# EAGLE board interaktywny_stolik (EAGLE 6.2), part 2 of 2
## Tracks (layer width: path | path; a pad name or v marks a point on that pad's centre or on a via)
0V
  Bottom 0.406: IC1.10 18.34,221.93 18.34,220.46 | 18.34,220.46 20.85,220.46 20.85,220.48 | 20.85,220.48 IC1.12 | IC1.5 18.34,216.1 18.34,220.46 | IC1.1 IC1.2 | IC1.2 22.07,216.1 22.07,220.48 20.85,220.48 | R6.2 20.96,211.69 20.96,214.41 22.12,214.41 IC1.2
0V1
  Bottom 0.406: IC2.10 98.34,221.93 98.34,220.46 | 98.34,220.46 100.85,220.46 100.85,220.48 | 100.85,220.48 IC2.12 | IC2.5 98.34,216.1 98.34,220.46 | IC2.1 IC2.2 | IC2.2 102.07,216.1 102.07,220.48 100.85,220.48 | R18.2 100.96,211.69 100.96,214.41 102.12,214.41 IC2.2
0V2
  Bottom 0.406: IC3.10 178.34,221.93 178.34,220.46 | 178.34,220.46 180.85,220.46 180.85,220.48 | 180.85,220.48 IC3.12 | IC3.5 178.34,216.1 178.34,220.46 | IC3.1 IC3.2 | IC3.2 182.07,216.1 182.07,220.48 180.85,220.48 | R30.2 180.96,211.69 180.96,214.41 182.12,214.41 IC3.2
0V3
  Bottom 0.406: IC4.10 18.34,141.93 18.34,140.46 | 18.34,140.46 20.85,140.46 20.85,140.48 | 20.85,140.48 IC4.12 | IC4.5 18.34,136.1 18.34,140.46 | IC4.1 IC4.2 | IC4.2 22.07,136.1 22.07,140.48 20.85,140.48 | R42.2 20.96,131.69 20.96,134.41 22.12,134.41 IC4.2
0V4
  Bottom 0.406: IC5.10 98.34,141.93 98.34,140.46 | 98.34,140.46 100.85,140.46 100.85,140.48 | 100.85,140.48 IC5.12 | IC5.5 98.34,136.1 98.34,140.46 | IC5.1 IC5.2 | IC5.2 102.07,136.1 102.07,140.48 100.85,140.48 | R54.2 100.96,131.69 100.96,134.41 102.12,134.41 IC5.2
0V5
  Bottom 0.406: IC6.10 178.34,141.93 178.34,140.46 | 178.34,140.46 180.85,140.46 180.85,140.48 | 180.85,140.48 IC6.12 | IC6.5 178.34,136.1 178.34,140.46 | IC6.1 IC6.2 | IC6.2 182.07,136.1 182.07,140.48 180.85,140.48 | R66.2 180.96,131.69 180.96,134.41 182.12,134.41 IC6.2
0V6
  Bottom 0.406: IC7.10 18.34,61.93 18.34,60.46 | 18.34,60.46 20.85,60.46 20.85,60.48 | 20.85,60.48 IC7.12 | IC7.5 18.34,56.1 18.34,60.46 | IC7.1 IC7.2 | IC7.2 22.07,56.1 22.07,60.48 20.85,60.48 | R78.2 20.96,51.69 20.96,54.41 22.12,54.41 IC7.2
0V7
  Bottom 0.406: IC8.10 98.34,61.93 98.34,60.46 | 98.34,60.46 100.85,60.46 100.85,60.48 | 100.85,60.48 IC8.12 | IC8.5 98.34,56.1 98.34,60.46 | IC8.1 IC8.2 | IC8.2 102.07,56.1 102.07,60.48 100.85,60.48 | R90.2 100.96,51.69 100.96,54.41 102.12,54.41 IC8.2
0V8
  Bottom 0.406: IC9.10 178.34,61.93 178.34,60.46 | 178.34,60.46 180.85,60.46 180.85,60.48 | 180.85,60.48 IC9.12 | IC9.5 178.34,56.1 178.34,60.46 | IC9.1 IC9.2 | IC9.2 182.07,56.1 182.07,60.48 180.85,60.48 | R102.2 180.96,51.69 180.96,54.41 182.12,54.41 IC9.2
GND  (via drill 0.6 pad 0.81)
  Top 0.406: v19.63,223.99 9.5,223.99 v9.47,223.96
  Top 0.813: v35.2,223.91 19.76,223.91 v19.63,223.96
  Bottom 0.406: IC1.11 19.63,221.93 19.63,222.06 | 19.61,224.01 v19.63,223.99
  Bottom 0.813: 40.95,203.39 41.02,203.39 41.02,220.58 35.2,220.58 v35.2,223.91 | v19.63,223.96 19.61,224.01 IC1.11
  Bottom 1.016: R2.1 9.47,223.83 v9.47,223.96 9.47,229.07 11.43,229.07 LED6.K | LED21.K 41,203.41 | 40.97,203.41 40.97,203.57 41,203.57 41,203.41 | 41,203.41 40.97,203.41 | 40.97,203.41 40.97,203.24 40.95,203.24 40.95,203.39
GND1  (via drill 0.6 pad 0.81)
  Top 0.406: v99.63,223.99 89.5,223.99 v89.47,223.96
  Top 0.813: v115.2,223.91 99.76,223.91 v99.63,223.96
  Bottom 0.406: IC2.11 99.63,221.93 99.63,222.06 | 99.61,224.01 v99.63,223.99
  Bottom 0.813: 120.95,203.39 121.02,203.39 121.02,220.58 115.2,220.58 v115.2,223.91 | v99.63,223.96 99.61,224.01 IC2.11
  Bottom 1.016: R14.1 89.47,223.83 v89.47,223.96 89.47,229.07 91.43,229.07 LED34.K | LED28.K 121,203.41 | 120.97,203.41 120.97,203.57 121,203.57 121,203.41 | 121,203.41 120.97,203.41 | 120.97,203.41 120.97,203.24 120.95,203.24 120.95,203.39
GND2  (via drill 0.6 pad 0.81)
  Top 0.406: v179.63,223.99 169.5,223.99 v169.47,223.96
  Top 0.813: v195.2,223.91 179.76,223.91 v179.63,223.96
  Bottom 0.406: IC3.11 179.63,221.93 179.63,222.06 | 179.61,224.01 v179.63,223.99
  Bottom 0.813: 200.95,203.39 201.02,203.39 201.02,220.58 195.2,220.58 v195.2,223.91 | v179.63,223.96 179.61,224.01 IC3.11
  Bottom 1.016: R26.1 169.47,223.83 v169.47,223.96 169.47,229.07 171.43,229.07 LED51.K | LED45.K 201,203.41 | 200.97,203.41 200.97,203.57 201,203.57 201,203.41 | 201,203.41 200.97,203.41 | 200.97,203.41 200.97,203.24 200.95,203.24 200.95,203.39
GND3  (via drill 0.6 pad 0.81)
  Top 0.406: v19.63,143.99 9.5,143.99 v9.47,143.96
  Top 0.813: v35.2,143.91 19.76,143.91 v19.63,143.96
  Bottom 0.406: IC4.11 19.63,141.93 19.63,142.06 | 19.61,144.01 v19.63,143.99
  Bottom 0.813: 40.95,123.39 41.02,123.39 41.02,140.58 35.2,140.58 v35.2,143.91 | v19.63,143.96 19.61,144.01 IC4.11
  Bottom 1.016: R38.1 9.47,143.83 v9.47,143.96 9.47,149.07 11.43,149.07 LED68.K | LED62.K 41,123.41 | 40.97,123.41 40.97,123.57 41,123.57 41,123.41 | 41,123.41 40.97,123.41 | 40.97,123.41 40.97,123.24 40.95,123.24 40.95,123.39
GND4  (via drill 0.6 pad 0.81)
  Top 0.406: v99.63,143.99 89.5,143.99 v89.47,143.96
  Top 0.813: v115.2,143.91 99.76,143.91 v99.63,143.96
  Bottom 0.406: IC5.11 99.63,141.93 99.63,142.06 | 99.61,144.01 v99.63,143.99
  Bottom 0.813: 120.95,123.39 121.02,123.39 121.02,140.58 115.2,140.58 v115.2,143.91 | v99.63,143.96 99.61,144.01 IC5.11
  Bottom 1.016: R50.1 89.47,143.83 v89.47,143.96 89.47,149.07 91.43,149.07 LED85.K | LED79.K 121,123.41 | 120.97,123.41 120.97,123.57 121,123.57 121,123.41 | 121,123.41 120.97,123.41 | 120.97,123.41 120.97,123.24 120.95,123.24 120.95,123.39
GND5  (via drill 0.6 pad 0.81)
  Top 0.406: v179.63,143.99 169.5,143.99 v169.47,143.96
  Top 0.813: v195.2,143.91 179.76,143.91 v179.63,143.96
  Bottom 0.406: IC6.11 179.63,141.93 179.63,142.06 | 179.61,144.01 v179.63,143.99
  Bottom 0.813: 200.95,123.39 201.02,123.39 201.02,140.58 195.2,140.58 v195.2,143.91 | v179.63,143.96 179.61,144.01 IC6.11
  Bottom 1.016: R62.1 169.47,143.83 v169.47,143.96 169.47,149.07 171.43,149.07 LED102.K | LED96.K 201,123.41 | 200.97,123.41 200.97,123.57 201,123.57 201,123.41 | 201,123.41 200.97,123.41 | 200.97,123.41 200.97,123.24 200.95,123.24 200.95,123.39
GND6  (via drill 0.6 pad 0.81)
  Top 0.406: v19.63,63.99 9.5,63.99 v9.47,63.96
  Top 0.813: v35.2,63.91 19.76,63.91 v19.63,63.96
  Bottom 0.406: IC7.11 19.63,61.93 19.63,62.06 | 19.61,64.01 v19.63,63.99
  Bottom 0.813: 40.95,43.39 41.02,43.39 41.02,60.58 35.2,60.58 v35.2,63.91 | v19.63,63.96 19.61,64.01 IC7.11
  Bottom 1.016: R74.1 9.47,63.83 v9.47,63.96 9.47,69.07 11.43,69.07 LED119.K | LED113.K 41,43.41 | 40.97,43.41 40.97,43.57 41,43.57 41,43.41 | 41,43.41 40.97,43.41 | 40.97,43.41 40.97,43.24 40.95,43.24 40.95,43.39
GND7  (via drill 0.6 pad 0.81)
  Top 0.406: v99.63,63.99 89.5,63.99 v89.47,63.96
  Top 0.813: v115.2,63.91 99.76,63.91 v99.63,63.96
  Bottom 0.406: IC8.11 99.63,61.93 99.63,62.06 | 99.61,64.01 v99.63,63.99
  Bottom 0.813: 120.95,43.39 121.02,43.39 121.02,60.58 115.2,60.58 v115.2,63.91 | v99.63,63.96 99.61,64.01 IC8.11
  Bottom 1.016: R86.1 89.47,63.83 v89.47,63.96 89.47,69.07 91.43,69.07 LED136.K | LED130.K 121,43.41 | 120.97,43.41 120.97,43.57 121,43.57 121,43.41 | 121,43.41 120.97,43.41 | 120.97,43.41 120.97,43.24 120.95,43.24 120.95,43.39
GND8  (via drill 0.6 pad 0.81)
  Top 0.406: v179.63,63.99 169.5,63.99 v169.47,63.96
  Top 0.813: v195.2,63.91 179.76,63.91 v179.63,63.96
  Bottom 0.406: IC9.11 179.63,61.93 179.63,62.06 | 179.61,64.01 v179.63,63.99
  Bottom 0.813: 200.95,43.39 201.02,43.39 201.02,60.58 195.2,60.58 v195.2,63.91 | v179.63,63.96 179.61,64.01 IC9.11
  Bottom 1.016: R98.1 169.47,63.83 v169.47,63.96 169.47,69.07 171.43,69.07 LED153.K | LED147.K 201,43.41 | 200.97,43.41 200.97,43.57 201,43.57 201,43.41 | 201,43.41 200.97,43.41 | 200.97,43.41 200.97,43.24 200.95,43.24 200.95,43.39
N$1  (via drill 0.6 pad 0.81)
  Top 0.406: v19.66,213.95 v13.31,213.95
  Bottom 0.406: 9.73,217.1 9.73,217.26 R1.1 12.73,213.95 v13.31,213.95 | IC1.3 20.83,216.1 20.83,216.16 20.85,216.16 20.85,215.15 20.63,215.15 19.71,214.23 19.71,214.01 v19.66,213.95
  Bottom 1.016: R2.2 R1.1
N$2
  Bottom 0.406: IC1.6 17.04,213.9 18.09,213.9 18.09,211.47 R3.2 17.42,211.47 17.4,205.57 25.35,205.6 25.37,211.47 23.67,211.44 R4.1
N$3
  Bottom 0.406: R3.1 14.53,213.14 15.8,213.14 15.8,216.1 IC1.7 15.77,216.11 11.48,216.11 11.48,224.06 R7.2
N$4  (via drill 0.6 pad 0.81)
  Top 0.813: v24.97,198.82 36.32,198.82 v36.32,198.84
  Bottom 0.406: R6.1 20.88,208.62 R4.2 23.47,208.62 23.47,208.37 | 22.45,208.82 22.35,208.82 22.35,213.62 26.11,213.62 26.11,204 24.92,204 24.92,198.79
  Bottom 0.813: 24.92,198.79 24.97,198.79 v24.97,198.82 | v36.32,198.84 38.46,198.84 T1.E
  Bottom 1.016: T1.E 38.56,198.82 38.56,198.66 | R4.2 20.9,208.75 20.9,208.82 22.45,208.82
N$5
  Bottom 1.016: R5.2 41,194.93 T1.C
N$6
  Bottom 0.406: R8.1 17.04,217.84 IC1.9 17.04,223.96 18.24,223.96 18.24,225.66 C2.2
N$7
  Bottom 0.406: R8.2 13.39,220.69 13.39,220 15.85,220 15.85,221.93 IC1.8 15.75,221.93 C1.2 15.72,225.66 15.72,227.16 20.14,227.16 20.14,230.52 24.64,230.52 R10.2
N$8
  Bottom 0.406: R10.1 21.74,229.02 R11.2 22.12,225.69 IC1.13
N$9
  Bottom 1.016: R7.1 13.21,226.91 13.21,228.66 C1.1 C2.1
N$10
  Bottom 0.406: IC1.14 23.42,221.93 23.42,225.69 R11.1
  Bottom 0.61: 55.22,235.57 30.15,235.57 30.15,228.64 27.23,228.64 27.23,225.56 24.59,225.56 R11.1
  Bottom 0.813: R12.2 55.22,195.51 55.22,235.57
N$11
  Bottom 0.61: 30.4,194.42 30.18,194.42 30.18,187.21
  Bottom 1.016: 31.42,210.7 LED1.A 31.6,210.7 31.6,204.35 30.4,204.35 30.4,194.42 | 30.18,187.21 31.42,187.21 LED20.K
N$12
  Bottom 0.61: 31.32,215.02 30.15,215.02 30.15,208.04
  Bottom 1.016: LED2.K 31.32,230.74 31.32,215.02 | 30.15,208.04 28.9,208.04 LED11.A
N$13
  Bottom 1.016: LED3.A 27.31,190.69 27.31,210.35 28.91,210.35 LED1.K
N$14
  Bottom 1.016: LED4.K 4.9,170.7 4.9,232.9 28.92,232.9 LED2.A
N$15
  Bottom 0.61: 11.38,193.91 10.19,193.91 10.19,186.12
  Bottom 1.016: LED5.K 11.38,210.72 11.38,193.91 | 10.19,186.12 11.47,186.12 LED4.A
N$16
  Bottom 1.016: LED3.K 7.01,190.59 7.01,230.72 LED6.A
N$17
  Bottom 1.016: R13.2 38.48,206.87 LED21.A
N$18  (via drill 0.6 pad 0.81)
  Top 0.406: v99.66,213.95 v93.31,213.95
  Bottom 0.406: 89.73,217.1 89.73,217.26 R9.1 92.73,213.95 v93.31,213.95 | IC2.3 100.83,216.1 100.83,216.16 100.85,216.16 100.85,215.15 100.63,215.15 99.71,214.23 99.71,214.01 v99.66,213.95
  Bottom 1.016: R14.2 R9.1
N$19
  Bottom 0.406: IC2.6 97.04,213.9 98.09,213.9 98.09,211.47 R15.2 97.42,211.47 97.4,205.57 105.35,205.6 105.37,211.47 103.67,211.44 R16.1
N$20
  Bottom 0.406: R15.1 94.53,213.14 95.8,213.14 95.8,216.1 IC2.7 95.77,216.11 91.48,216.11 91.48,224.06 R19.2
N$21  (via drill 0.6 pad 0.81)
  Top 0.813: v104.97,198.82 116.32,198.82 v116.32,198.84
  Bottom 0.406: R18.1 100.88,208.62 R16.2 103.47,208.62 103.47,208.37 | 102.45,208.82 102.35,208.82 102.35,213.62 106.11,213.62 106.11,204 104.92,204 104.92,198.79
  Bottom 0.813: 104.92,198.79 104.97,198.79 v104.97,198.82 | v116.32,198.84 118.46,198.84 T2.E
  Bottom 1.016: T2.E 118.56,198.82 118.56,198.66 | R16.2 100.9,208.75 100.9,208.82 102.45,208.82
N$22
  Bottom 0.61: 50.44,229.04 50.27,229.04 50.27,232.67
  Bottom 1.016: LED12.A 48.69,210.75 48.69,213.17 50.44,213.17 50.44,229.04 | 50.27,232.67 50.47,232.67 50.47,233.51 33.25,233.51 33.25,214.77 33.35,214.77 33.35,203.13 32.61,203.13 32.61,202.65 32.06,202.65 32.06,190.56 31.44,190.56 LED11.K
N$23
  Bottom 0.61: 51.16,193.43 50.19,193.43 50.19,187.74
  Bottom 1.016: LED12.K 51.16,210.75 51.16,193.43 | 50.19,187.74 51.47,187.74 LED13.A
N$24
  Bottom 1.016: LED13.K 48.9,170.68 48.9,166.51 74.96,166.51 74.96,232.5 68.93,232.5 LED14.A
N$25
  Bottom 1.016: LED14.K 73.46,230.74 73.46,190.66 71.46,190.66 LED15.A
N$26
  Bottom 1.016: LED16.A 68.94,190.72 LED15.K 68.92,195.51 R12.1
N$27
  Bottom 0.61: 71.5,186.67 70.23,186.67 70.23,193.2
  Bottom 1.016: 71.48,210.7 LED17.A 71.45,193.2 70.23,193.2 | LED16.K 71.5,170.75 71.5,186.67
N$28
  Bottom 0.61: 49.96,173.72 50.22,173.72 50.22,167.68 67.44,167.68 67.49,203.26
  Bottom 1.016: LED18.A 48.77,190.69 48.77,185.35 49.96,185.35 49.96,173.72 | 67.49,203.26 68.91,203.34 LED17.K
N$29
  Bottom 1.016: 51.44,230.69 LED19.A 53.14,230.69 53.14,190.84 51.44,190.84 LED18.K
N$30
  Bottom 1.016: LED20.A 28.75,170.75 28.75,168.46 46.69,168.46 46.69,215.61 48.92,215.61 LED19.K
N$31
  Bottom 1.016: R17.2 121,194.93 T2.C
N$32
  Bottom 0.406: R20.1 97.04,217.84 IC2.9 97.04,223.96 98.24,223.96 98.24,225.66 C4.2
N$33
  Bottom 0.406: R20.2 93.39,220.69 93.39,220 95.85,220 95.85,221.93 IC2.8 95.75,221.93 C3.2 95.72,225.66 95.72,227.16 100.14,227.16 100.14,230.52 104.64,230.52 R21.2
N$34
  Bottom 1.016: R19.1 93.21,226.91 93.21,228.66 C3.1 C4.1
N$35
  Bottom 0.406: R21.1 101.74,229.02 R22.2 102.12,225.69 IC2.13
N$36
  Bottom 0.406: IC2.14 103.42,221.93 103.42,225.69 R22.1
  Bottom 0.61: 135.22,235.57 110.15,235.57 110.15,228.64 107.23,228.64 107.23,225.56 104.59,225.56 R22.1
  Bottom 0.813: R23.2 135.22,195.51 135.22,235.57
N$37
  Bottom 0.61: 130.44,229.04 130.27,229.04 130.27,232.67
  Bottom 1.016: LED8.A 128.69,210.75 128.69,213.17 130.44,213.17 130.44,229.04 | 130.27,232.67 130.47,232.67 130.47,233.51 113.25,233.51 113.25,214.77 113.35,214.77 113.35,203.13 112.61,203.13 112.61,202.65 112.06,202.65 112.06,190.56 111.44,190.56 LED7.K
N$38
  Bottom 0.61: 131.16,193.43 130.19,193.43 130.19,187.74
  Bottom 1.016: LED8.K 131.16,210.75 131.16,193.43 | 130.19,187.74 131.47,187.74 LED9.A
N$39
  Bottom 1.016: LED9.K 128.9,170.68 128.9,166.51 154.96,166.51 154.96,232.5 148.93,232.5 LED10.A
N$40
  Bottom 1.016: LED10.K 153.46,230.74 153.46,190.66 151.46,190.66 LED22.A
N$41
  Bottom 1.016: LED23.A 148.94,190.72 LED22.K R23.1
N$42
  Bottom 0.61: 151.5,186.67 150.23,186.67 150.23,193.2
  Bottom 1.016: 151.48,210.7 LED24.A 151.45,193.2 150.23,193.2 | LED23.K 151.5,170.75 151.5,186.67
N$43
  Bottom 0.61: 129.96,173.72 130.22,173.72 130.22,167.68 147.44,167.68 147.49,203.26
  Bottom 1.016: LED25.A 128.77,190.69 128.77,185.35 129.96,185.35 129.96,173.72 | 147.49,203.26 148.91,203.34 LED24.K
N$44
  Bottom 1.016: 131.44,230.69 LED26.A 133.14,230.69 133.14,190.84 131.44,190.84 LED25.K
N$45
  Bottom 1.016: LED27.A 108.75,170.75 108.75,168.46 126.69,168.46 126.69,215.61 128.92,215.61 LED26.K
N$46
  Bottom 0.61: 110.4,194.42 110.18,194.42 110.18,187.21
  Bottom 1.016: 111.42,210.7 LED29.A 111.6,210.7 111.6,204.35 110.4,204.35 110.4,194.42 | 110.18,187.21 111.42,187.21 LED27.K
N$47
  Bottom 0.61: 111.32,215.02 110.15,215.02 110.15,208.04
  Bottom 1.016: LED30.K 111.32,230.74 111.32,215.02 | 110.15,208.04 108.9,208.04 LED7.A
N$48
  Bottom 1.016: LED31.A 107.31,190.69 107.31,210.35 108.91,210.35 LED29.K
N$49
  Bottom 1.016: LED32.K 84.9,170.7 84.9,232.9 108.92,232.9 LED30.A
N$50
  Bottom 0.61: 91.38,193.91 90.19,193.91 90.19,186.12
  Bottom 1.016: LED33.K 91.38,210.72 91.38,193.91 | 90.19,186.12 91.47,186.12 LED32.A
N$51
  Bottom 1.016: LED31.K 87.01,190.59 87.01,230.72 LED34.A
N$52
  Bottom 1.016: R24.2 118.48,206.87 LED28.A
N$53  (via drill 0.6 pad 0.81)
  Top 0.406: v179.66,213.95 v173.31,213.95
  Bottom 0.406: 169.73,217.1 169.73,217.26 R25.1 172.73,213.95 v173.31,213.95 | IC3.3 180.83,216.1 180.83,216.16 180.85,216.16 180.85,215.15 180.63,215.15 179.71,214.23 179.71,214.01 v179.66,213.95
  Bottom 1.016: R26.2 R25.1
N$54
  Bottom 0.406: IC3.6 177.04,213.9 178.09,213.9 178.09,211.47 R27.2 177.42,211.47 177.4,205.57 185.35,205.6 185.37,211.47 183.67,211.44 R28.1
N$55
  Bottom 0.406: R27.1 174.53,213.14 175.8,213.14 175.8,216.1 IC3.7 175.77,216.11 171.48,216.11 171.48,224.06 R31.2
N$56  (via drill 0.6 pad 0.81)
  Top 0.813: v184.97,198.82 196.32,198.82 v196.32,198.84
  Bottom 0.406: R30.1 180.88,208.62 R28.2 183.47,208.62 183.47,208.37 | 182.45,208.82 182.35,208.82 182.35,213.62 186.11,213.62 186.11,204 184.92,204 184.92,198.79
  Bottom 0.813: 184.92,198.79 184.97,198.79 v184.97,198.82 | v196.32,198.84 198.46,198.84 T3.E
  Bottom 1.016: T3.E 198.56,198.82 198.56,198.66 | R28.2 180.9,208.75 180.9,208.82 182.45,208.82
N$57
  Bottom 1.016: R29.2 201,194.93 T3.C
N$58
  Bottom 0.406: R32.1 177.04,217.84 IC3.9 177.04,223.96 178.24,223.96 178.24,225.66 C6.2
N$59
  Bottom 0.406: R32.2 173.39,220.69 173.39,220 175.85,220 175.85,221.93 IC3.8 175.75,221.93 C5.2 175.72,225.66 175.72,227.16 180.14,227.16 180.14,230.52 184.64,230.52 R33.2
N$60
  Bottom 1.016: R31.1 173.21,226.91 173.21,228.66 C5.1 C6.1
N$61
  Bottom 0.406: R33.1 181.74,229.02 R34.2 182.12,225.69 IC3.13
N$62
  Bottom 0.406: IC3.14 183.42,221.93 183.42,225.69 R34.1
  Bottom 0.61: 215.22,235.57 190.15,235.57 190.15,228.64 187.23,228.64 187.23,225.56 184.59,225.56 R34.1
  Bottom 0.813: R35.2 215.22,195.51 215.22,235.57
N$63
  Bottom 0.61: 210.44,229.04 210.27,229.04 210.27,232.67
  Bottom 1.016: LED36.A 208.69,210.75 208.69,213.17 210.44,213.17 210.44,229.04 | 210.27,232.67 210.47,232.67 210.47,233.51 193.25,233.51 193.25,214.77 193.35,214.77 193.35,203.13 192.61,203.13 192.61,202.65 192.06,202.65 192.06,190.56 191.44,190.56 LED35.K
N$64
  Bottom 0.61: 211.16,193.43 210.19,193.43 210.19,187.74
  Bottom 1.016: LED36.K 211.16,210.75 211.16,193.43 | 210.19,187.74 211.47,187.74 LED37.A
N$65
  Bottom 1.016: LED37.K 208.9,170.68 208.9,166.51 234.96,166.51 234.96,232.5 228.93,232.5 LED38.A
N$66
  Bottom 1.016: LED38.K 233.46,230.74 233.46,190.66 231.46,190.66 LED39.A
N$67
  Bottom 1.016: LED40.A 228.94,190.72 LED39.K R35.1
N$68
  Bottom 0.61: 231.5,186.67 230.23,186.67 230.23,193.2
  Bottom 1.016: 231.48,210.7 LED41.A 231.45,193.2 230.23,193.2 | LED40.K 231.5,170.75 231.5,186.67
N$69
  Bottom 0.61: 209.96,173.72 210.22,173.72 210.22,167.68 227.44,167.68 227.49,203.26
  Bottom 1.016: LED42.A 208.77,190.69 208.77,185.35 209.96,185.35 209.96,173.72 | 227.49,203.26 228.91,203.34 LED41.K
N$70
  Bottom 1.016: 211.44,230.69 LED43.A 213.14,230.69 213.14,190.84 211.44,190.84 LED42.K
N$71
  Bottom 1.016: LED44.A 188.75,170.75 188.75,168.46 206.69,168.46 206.69,215.61 208.92,215.61 LED43.K
N$72
  Bottom 0.61: 190.4,194.42 190.18,194.42 190.18,187.21
  Bottom 1.016: 191.42,210.7 LED46.A 191.6,210.7 191.6,204.35 190.4,204.35 190.4,194.42 | 190.18,187.21 191.42,187.21 LED44.K
N$73
  Bottom 0.61: 191.32,215.02 190.15,215.02 190.15,208.04
  Bottom 1.016: LED47.K 191.32,230.74 191.32,215.02 | 190.15,208.04 188.9,208.04 LED35.A
N$74
  Bottom 1.016: LED48.A 187.31,190.69 187.31,210.35 188.91,210.35 LED46.K
N$75
  Bottom 1.016: LED49.K 164.9,170.7 164.9,232.9 188.92,232.9 LED47.A
N$76
  Bottom 0.61: 171.38,193.91 170.19,193.91 170.19,186.12
  Bottom 1.016: LED50.K 171.38,210.72 171.38,193.91 | 170.19,186.12 171.47,186.12 LED49.A
N$77
  Bottom 1.016: LED48.K 167.01,190.59 167.01,230.72 LED51.A
N$78
  Bottom 1.016: R36.2 198.48,206.87 LED45.A
N$79  (via drill 0.6 pad 0.81)
  Top 0.406: v19.66,133.95 v13.31,133.95
  Bottom 0.406: 9.73,137.1 9.73,137.26 R37.1 12.73,133.95 v13.31,133.95 | IC4.3 20.83,136.1 20.83,136.16 20.85,136.16 20.85,135.15 20.63,135.15 19.71,134.23 19.71,134.01 v19.66,133.95
  Bottom 1.016: R38.2 R37.1
N$80
  Bottom 0.406: IC4.6 17.04,133.9 18.09,133.9 18.09,131.47 R39.2 17.42,131.47 17.4,125.57 25.35,125.6 25.37,131.47 23.67,131.44 R40.1
N$81
  Bottom 0.406: R39.1 14.53,133.14 15.8,133.14 15.8,136.1 IC4.7 15.77,136.11 11.48,136.11 11.48,144.06 R43.2
N$82  (via drill 0.6 pad 0.81)
  Top 0.813: v24.97,118.82 36.32,118.82 v36.32,118.84
  Bottom 0.406: R42.1 20.88,128.62 R40.2 23.47,128.62 23.47,128.37 | 22.45,128.82 22.35,128.82 22.35,133.62 26.11,133.62 26.11,124 24.92,124 24.92,118.79
  Bottom 0.813: 24.92,118.79 24.97,118.79 v24.97,118.82 | v36.32,118.84 38.46,118.84 T4.E
  Bottom 1.016: T4.E 38.56,118.82 38.56,118.66 | R40.2 20.9,128.75 20.9,128.82 22.45,128.82
N$83
  Bottom 1.016: R41.2 41,114.93 T4.C
N$84
  Bottom 0.406: R44.1 17.04,137.84 IC4.9 17.04,143.96 18.24,143.96 18.24,145.66 C8.2
N$85
  Bottom 0.406: R44.2 13.39,140.69 13.39,140 15.85,140 15.85,141.93 IC4.8 15.75,141.93 C7.2 15.72,145.66 15.72,147.16 20.14,147.16 20.14,150.52 24.64,150.52 R45.2
N$86
  Bottom 1.016: R43.1 13.21,146.91 13.21,148.66 C7.1 C8.1
N$87
  Bottom 0.406: R45.1 21.74,149.02 R46.2 22.12,145.69 IC4.13
N$88
  Bottom 0.406: IC4.14 23.42,141.93 23.42,145.69 R46.1
  Bottom 0.61: 55.22,155.57 30.15,155.57 30.15,148.64 27.23,148.64 27.23,145.56 24.59,145.56 R46.1
  Bottom 0.813: R47.2 55.22,115.51 55.22,155.57
N$89
  Bottom 0.61: 50.44,149.04 50.27,149.04 50.27,152.67
  Bottom 1.016: LED53.A 48.69,130.75 48.69,133.17 50.44,133.17 50.44,149.04 | 50.27,152.67 50.47,152.67 50.47,153.51 33.25,153.51 33.25,134.77 33.35,134.77 33.35,123.13 32.61,123.13 32.61,122.65 32.06,122.65 32.06,110.56 31.44,110.56 LED52.K
N$90
  Bottom 0.61: 51.16,113.43 50.19,113.43 50.19,107.74
  Bottom 1.016: LED53.K 51.16,130.75 51.16,113.43 | 50.19,107.74 51.47,107.74 LED54.A
N$91
  Bottom 1.016: LED54.K 48.9,90.68 48.9,86.51 74.96,86.51 74.96,152.5 68.93,152.5 LED55.A
N$92
  Bottom 1.016: LED55.K 73.46,150.74 73.46,110.66 71.46,110.66 LED56.A
N$93
  Bottom 1.016: LED57.A 68.94,110.72 LED56.K 68.92,115.51 R47.1
N$94
  Bottom 0.61: 71.5,106.67 70.23,106.67 70.23,113.2
  Bottom 1.016: 71.48,130.7 LED58.A 71.45,113.2 70.23,113.2 | LED57.K 71.5,90.75 71.5,106.67
N$95
  Bottom 0.61: 49.96,93.72 50.22,93.72 50.22,87.68 67.44,87.68 67.49,123.26
  Bottom 1.016: LED59.A 48.77,110.69 48.77,105.35 49.96,105.35 49.96,93.72 | 67.49,123.26 68.91,123.34 LED58.K
N$96
  Bottom 1.016: 51.44,150.69 LED60.A 53.14,150.69 53.14,110.84 51.44,110.84 LED59.K
N$97
  Bottom 1.016: LED61.A 28.75,90.75 28.75,88.46 46.69,88.46 46.69,135.61 48.92,135.61 LED60.K
N$98
  Bottom 0.61: 30.4,114.42 30.18,114.42 30.18,107.21
  Bottom 1.016: 31.42,130.7 LED63.A 31.6,130.7 31.6,124.35 30.4,124.35 30.4,114.42 | 30.18,107.21 31.42,107.21 LED61.K
N$99
  Bottom 0.61: 31.32,135.02 30.15,135.02 30.15,128.04
  Bottom 1.016: LED64.K 31.32,150.74 31.32,135.02 | 30.15,128.04 28.9,128.04 LED52.A
N$100
  Bottom 1.016: LED65.A 27.31,110.69 27.31,130.35 28.91,130.35 LED63.K
N$101
  Bottom 1.016: LED66.K 4.9,90.7 4.9,152.9 28.92,152.9 LED64.A
N$102
  Bottom 0.61: 11.38,113.91 10.19,113.91 10.19,106.12
  Bottom 1.016: LED67.K 11.38,130.72 11.38,113.91 | 10.19,106.12 11.47,106.12 LED66.A
N$103
  Bottom 1.016: LED65.K 7.01,110.59 7.01,150.72 LED68.A
N$104
  Bottom 1.016: R48.2 38.48,126.87 LED62.A
N$105  (via drill 0.6 pad 0.81)
  Top 0.406: v99.66,133.95 v93.31,133.95
  Bottom 0.406: 89.73,137.1 89.73,137.26 R49.1 92.73,133.95 v93.31,133.95 | IC5.3 100.83,136.1 100.83,136.16 100.85,136.16 100.85,135.15 100.63,135.15 99.71,134.23 99.71,134.01 v99.66,133.95
  Bottom 1.016: R50.2 R49.1
N$106
  Bottom 0.406: IC5.6 97.04,133.9 98.09,133.9 98.09,131.47 R51.2 97.42,131.47 97.4,125.57 105.35,125.6 105.37,131.47 103.67,131.44 R52.1
N$107
  Bottom 0.406: R51.1 94.53,133.14 95.8,133.14 95.8,136.1 IC5.7 95.77,136.11 91.48,136.11 91.48,144.06 R55.2
N$108  (via drill 0.6 pad 0.81)
  Top 0.813: v104.97,118.82 116.32,118.82 v116.32,118.84
  Bottom 0.406: R54.1 100.88,128.62 R52.2 103.47,128.62 103.47,128.37 | 102.45,128.82 102.35,128.82 102.35,133.62 106.11,133.62 106.11,124 104.92,124 104.92,118.79
  Bottom 0.813: 104.92,118.79 104.97,118.79 v104.97,118.82 | v116.32,118.84 118.46,118.84 T5.E
  Bottom 1.016: T5.E 118.56,118.82 118.56,118.66 | R52.2 100.9,128.75 100.9,128.82 102.45,128.82
N$109
  Bottom 1.016: R53.2 121,114.93 T5.C
N$110
  Bottom 0.406: R56.1 97.04,137.84 IC5.9 97.04,143.96 98.24,143.96 98.24,145.66 C10.2
N$111
  Bottom 0.406: R56.2 93.39,140.69 93.39,140 95.85,140 95.85,141.93 IC5.8 95.75,141.93 C9.2 95.72,145.66 95.72,147.16 100.14,147.16 100.14,150.52 104.64,150.52 R57.2
N$112
  Bottom 1.016: R55.1 93.21,146.91 93.21,148.66 C9.1 C10.1
N$113
  Bottom 0.406: R57.1 101.74,149.02 R58.2 102.12,145.69 IC5.13
N$114
  Bottom 0.406: IC5.14 103.42,141.93 103.42,145.69 R58.1
  Bottom 0.61: 135.22,155.57 110.15,155.57 110.15,148.64 107.23,148.64 107.23,145.56 104.59,145.56 R58.1
  Bottom 0.813: R59.2 135.22,115.51 135.22,155.57
N$115
  Bottom 0.61: 130.44,149.04 130.27,149.04 130.27,152.67
  Bottom 1.016: LED70.A 128.69,130.75 128.69,133.17 130.44,133.17 130.44,149.04 | 130.27,152.67 130.47,152.67 130.47,153.51 113.25,153.51 113.25,134.77 113.35,134.77 113.35,123.13 112.61,123.13 112.61,122.65 112.06,122.65 112.06,110.56 111.44,110.56 LED69.K
N$116
  Bottom 0.61: 131.16,113.43 130.19,113.43 130.19,107.74
  Bottom 1.016: LED70.K 131.16,130.75 131.16,113.43 | 130.19,107.74 131.47,107.74 LED71.A
N$117
  Bottom 1.016: LED71.K 128.9,90.68 128.9,86.51 154.96,86.51 154.96,152.5 148.93,152.5 LED72.A
N$118
  Bottom 1.016: LED72.K 153.46,150.74 153.46,110.66 151.46,110.66 LED73.A
N$119
  Bottom 1.016: LED74.A 148.94,110.72 LED73.K R59.1
N$120
  Bottom 0.61: 151.5,106.67 150.23,106.67 150.23,113.2
  Bottom 1.016: 151.48,130.7 LED75.A 151.45,113.2 150.23,113.2 | LED74.K 151.5,90.75 151.5,106.67
N$121
  Bottom 0.61: 129.96,93.72 130.22,93.72 130.22,87.68 147.44,87.68 147.49,123.26
  Bottom 1.016: LED76.A 128.77,110.69 128.77,105.35 129.96,105.35 129.96,93.72 | 147.49,123.26 148.91,123.34 LED75.K
N$122
  Bottom 1.016: 131.44,150.69 LED77.A 133.14,150.69 133.14,110.84 131.44,110.84 LED76.K
N$123
  Bottom 1.016: LED78.A 108.75,90.75 108.75,88.46 126.69,88.46 126.69,135.61 128.92,135.61 LED77.K
N$124
  Bottom 0.61: 110.4,114.42 110.18,114.42 110.18,107.21
  Bottom 1.016: 111.42,130.7 LED80.A 111.6,130.7 111.6,124.35 110.4,124.35 110.4,114.42 | 110.18,107.21 111.42,107.21 LED78.K
N$125
  Bottom 0.61: 111.32,135.02 110.15,135.02 110.15,128.04
  Bottom 1.016: LED81.K 111.32,150.74 111.32,135.02 | 110.15,128.04 108.9,128.04 LED69.A
N$126
  Bottom 1.016: LED82.A 107.31,110.69 107.31,130.35 108.91,130.35 LED80.K
N$127
  Bottom 1.016: LED83.K 84.9,90.7 84.9,152.9 108.92,152.9 LED81.A
N$128
  Bottom 0.61: 91.38,113.91 90.19,113.91 90.19,106.12
  Bottom 1.016: LED84.K 91.38,130.72 91.38,113.91 | 90.19,106.12 91.47,106.12 LED83.A
N$129
  Bottom 1.016: LED82.K 87.01,110.59 87.01,150.72 LED85.A
N$130
  Bottom 1.016: R60.2 118.48,126.87 LED79.A
N$131  (via drill 0.6 pad 0.81)
  Top 0.406: v179.66,133.95 v173.31,133.95
  Bottom 0.406: 169.73,137.1 169.73,137.26 R61.1 172.73,133.95 v173.31,133.95 | IC6.3 180.83,136.1 180.83,136.16 180.85,136.16 180.85,135.15 180.63,135.15 179.71,134.23 179.71,134.01 v179.66,133.95
  Bottom 1.016: R62.2 R61.1
N$132
  Bottom 0.406: IC6.6 177.04,133.9 178.09,133.9 178.09,131.47 R63.2 177.42,131.47 177.4,125.57 185.35,125.6 185.37,131.47 183.67,131.44 R64.1
N$133
  Bottom 0.406: R63.1 174.53,133.14 175.8,133.14 175.8,136.1 IC6.7 175.77,136.11 171.48,136.11 171.48,144.06 R67.2
N$134  (via drill 0.6 pad 0.81)
  Top 0.813: v184.97,118.82 196.32,118.82 v196.32,118.84
  Bottom 0.406: R66.1 180.88,128.62 R64.2 183.47,128.62 183.47,128.37 | 182.45,128.82 182.35,128.82 182.35,133.62 186.11,133.62 186.11,124 184.92,124 184.92,118.79
  Bottom 0.813: 184.92,118.79 184.97,118.79 v184.97,118.82 | v196.32,118.84 198.46,118.84 T6.E
  Bottom 1.016: T6.E 198.56,118.82 198.56,118.66 | R64.2 180.9,128.75 180.9,128.82 182.45,128.82
N$135
  Bottom 1.016: R65.2 201,114.93 T6.C
N$136
  Bottom 0.406: R68.1 177.04,137.84 IC6.9 177.04,143.96 178.24,143.96 178.24,145.66 C12.2
N$137
  Bottom 0.406: R68.2 173.39,140.69 173.39,140 175.85,140 175.85,141.93 IC6.8 175.75,141.93 C11.2 175.72,145.66 175.72,147.16 180.14,147.16 180.14,150.52 184.64,150.52 R69.2
N$138
  Bottom 1.016: R67.1 173.21,146.91 173.21,148.66 C11.1 C12.1
N$139
  Bottom 0.406: R69.1 181.74,149.02 R70.2 182.12,145.69 IC6.13
N$140
  Bottom 0.406: IC6.14 183.42,141.93 183.42,145.69 R70.1
  Bottom 0.61: 215.22,155.57 190.15,155.57 190.15,148.64 187.23,148.64 187.23,145.56 184.59,145.56 R70.1
  Bottom 0.813: R71.2 215.22,115.51 215.22,155.57
N$141
  Bottom 0.61: 210.44,149.04 210.27,149.04 210.27,152.67
  Bottom 1.016: LED87.A 208.69,130.75 208.69,133.17 210.44,133.17 210.44,149.04 | 210.27,152.67 210.47,152.67 210.47,153.51 193.25,153.51 193.25,134.77 193.35,134.77 193.35,123.13 192.61,123.13 192.61,122.65 192.06,122.65 192.06,110.56 191.44,110.56 LED86.K
N$142
  Bottom 0.61: 211.16,113.43 210.19,113.43 210.19,107.74
  Bottom 1.016: LED87.K 211.16,130.75 211.16,113.43 | 210.19,107.74 211.47,107.74 LED88.A
N$143
  Bottom 1.016: LED88.K 208.9,90.68 208.9,86.51 234.96,86.51 234.96,152.5 228.93,152.5 LED89.A
N$144
  Bottom 1.016: LED89.K 233.46,150.74 233.46,110.66 231.46,110.66 LED90.A
N$145
  Bottom 1.016: LED91.A 228.94,110.72 LED90.K R71.1
N$146
  Bottom 0.61: 231.5,106.67 230.23,106.67 230.23,113.2
  Bottom 1.016: 231.48,130.7 LED92.A 231.45,113.2 230.23,113.2 | LED91.K 231.5,90.75 231.5,106.67
N$147
  Bottom 0.61: 209.96,93.72 210.22,93.72 210.22,87.68 227.44,87.68 227.49,123.26
  Bottom 1.016: LED93.A 208.77,110.69 208.77,105.35 209.96,105.35 209.96,93.72 | 227.49,123.26 228.91,123.34 LED92.K
N$148
  Bottom 1.016: 211.44,150.69 LED94.A 213.14,150.69 213.14,110.84 211.44,110.84 LED93.K
N$149
  Bottom 1.016: LED95.A 188.75,90.75 188.75,88.46 206.69,88.46 206.69,135.61 208.92,135.61 LED94.K
N$150
  Bottom 0.61: 190.4,114.42 190.18,114.42 190.18,107.21
  Bottom 1.016: 191.42,130.7 LED97.A 191.6,130.7 191.6,124.35 190.4,124.35 190.4,114.42 | 190.18,107.21 191.42,107.21 LED95.K
N$151
  Bottom 0.61: 191.32,135.02 190.15,135.02 190.15,128.04
  Bottom 1.016: LED98.K 191.32,150.74 191.32,135.02 | 190.15,128.04 188.9,128.04 LED86.A
N$152
  Bottom 1.016: LED99.A 187.31,110.69 187.31,130.35 188.91,130.35 LED97.K
N$153
  Bottom 1.016: LED100.K 164.9,90.7 164.9,152.9 188.92,152.9 LED98.A
N$154
  Bottom 0.61: 171.38,113.91 170.19,113.91 170.19,106.12
  Bottom 1.016: LED101.K 171.38,130.72 171.38,113.91 | 170.19,106.12 171.47,106.12 LED100.A
N$155
  Bottom 1.016: LED99.K 167.01,110.59 167.01,150.72 LED102.A
N$156
  Bottom 1.016: R72.2 198.48,126.87 LED96.A
N$157  (via drill 0.6 pad 0.81)
  Top 0.406: v19.66,53.95 v13.31,53.95
  Bottom 0.406: 9.73,57.1 9.73,57.26 R73.1 12.73,53.95 v13.31,53.95 | IC7.3 20.83,56.1 20.83,56.16 20.85,56.16 20.85,55.15 20.63,55.15 19.71,54.23 19.71,54.01 v19.66,53.95
  Bottom 1.016: R74.2 R73.1
N$158
  Bottom 0.406: IC7.6 17.04,53.9 18.09,53.9 18.09,51.47 R75.2 17.42,51.47 17.4,45.57 25.35,45.6 25.37,51.47 23.67,51.44 R76.1
N$159
  Bottom 0.406: R75.1 14.53,53.14 15.8,53.14 15.8,56.1 IC7.7 15.77,56.11 11.48,56.11 11.48,64.06 R79.2
N$160  (via drill 0.6 pad 0.81)
  Top 0.813: v24.97,38.82 36.32,38.82 v36.32,38.84
  Bottom 0.406: R78.1 20.88,48.62 R76.2 23.47,48.62 23.47,48.37 | 22.45,48.82 22.35,48.82 22.35,53.62 26.11,53.62 26.11,44 24.92,44 24.92,38.79
  Bottom 0.813: 24.92,38.79 24.97,38.79 v24.97,38.82 | v36.32,38.84 38.46,38.84 T7.E
  Bottom 1.016: T7.E 38.56,38.82 38.56,38.66 | R76.2 20.9,48.75 20.9,48.82 22.45,48.82
N$161
  Bottom 1.016: R77.2 41,34.93 T7.C
N$162
  Bottom 0.406: R80.1 17.04,57.84 IC7.9 17.04,63.96 18.24,63.96 18.24,65.66 C14.2
N$163
  Bottom 0.406: R80.2 13.39,60.69 13.39,60 15.85,60 15.85,61.93 IC7.8 15.75,61.93 C13.2 15.72,65.66 15.72,67.16 20.14,67.16 20.14,70.52 24.64,70.52 R81.2
N$164
  Bottom 1.016: R79.1 13.21,66.91 13.21,68.66 C13.1 C14.1
N$165
  Bottom 0.406: R81.1 21.74,69.02 R82.2 22.12,65.69 IC7.13
N$166
  Bottom 0.406: IC7.14 23.42,61.93 23.42,65.69 R82.1
  Bottom 0.61: 55.22,75.57 30.15,75.57 30.15,68.64 27.23,68.64 27.23,65.56 24.59,65.56 R82.1
  Bottom 0.813: R83.2 55.22,35.51 55.22,75.57
N$167
  Bottom 0.61: 50.44,69.04 50.27,69.04 50.27,72.67
  Bottom 1.016: LED104.A 48.69,50.75 48.69,53.17 50.44,53.17 50.44,69.04 | 50.27,72.67 50.47,72.67 50.47,73.51 33.25,73.51 33.25,54.77 33.35,54.77 33.35,43.13 32.61,43.13 32.61,42.65 32.06,42.65 32.06,30.56 31.44,30.56 LED103.K
N$168
  Bottom 0.61: 51.16,33.43 50.19,33.43 50.19,27.74
  Bottom 1.016: LED104.K 51.16,50.75 51.16,33.43 | 50.19,27.74 51.47,27.74 LED105.A
N$169
  Bottom 1.016: LED105.K 48.9,10.68 48.9,6.51 74.96,6.51 74.96,72.5 68.93,72.5 LED106.A
N$170
  Bottom 1.016: LED106.K 73.46,70.74 73.46,30.66 71.46,30.66 LED107.A
N$171
  Bottom 1.016: LED108.A 68.94,30.72 LED107.K 68.92,35.51 R83.1
N$172
  Bottom 0.61: 71.5,26.67 70.23,26.67 70.23,33.2
  Bottom 1.016: 71.48,50.7 LED109.A 71.45,33.2 70.23,33.2 | LED108.K 71.5,10.75 71.5,26.67
N$173
  Bottom 0.61: 49.96,13.72 50.22,13.72 50.22,7.68 67.44,7.68 67.49,43.26
  Bottom 1.016: LED110.A 48.77,30.69 48.77,25.35 49.96,25.35 49.96,13.72 | 67.49,43.26 68.91,43.34 LED109.K
N$174
  Bottom 1.016: 51.44,70.69 LED111.A 53.14,70.69 53.14,30.84 51.44,30.84 LED110.K
N$175
  Bottom 1.016: LED112.A 28.75,10.75 28.75,8.46 46.69,8.46 46.69,55.61 48.92,55.61 LED111.K
N$176
  Bottom 0.61: 30.4,34.42 30.18,34.42 30.18,27.21
  Bottom 1.016: 31.42,50.7 LED114.A 31.6,50.7 31.6,44.35 30.4,44.35 30.4,34.42 | 30.18,27.21 31.42,27.21 LED112.K
N$177
  Bottom 0.61: 31.32,55.02 30.15,55.02 30.15,48.04
  Bottom 1.016: LED115.K 31.32,70.74 31.32,55.02 | 30.15,48.04 28.9,48.04 LED103.A
N$178
  Bottom 1.016: LED116.A 27.31,30.69 27.31,50.35 28.91,50.35 LED114.K
N$179
  Bottom 1.016: LED117.K 4.9,10.7 4.9,72.9 28.92,72.9 LED115.A
N$180
  Bottom 0.61: 11.38,33.91 10.19,33.91 10.19,26.12
  Bottom 1.016: LED118.K 11.38,50.72 11.38,33.91 | 10.19,26.12 11.47,26.12 LED117.A
N$181
  Bottom 1.016: LED116.K 7.01,30.59 7.01,70.72 LED119.A
N$182
  Bottom 1.016: R84.2 38.48,46.87 LED113.A
N$183  (via drill 0.6 pad 0.81)
  Top 0.406: v99.66,53.95 v93.31,53.95
  Bottom 0.406: 89.73,57.1 89.73,57.26 R85.1 92.73,53.95 v93.31,53.95 | IC8.3 100.83,56.1 100.83,56.16 100.85,56.16 100.85,55.15 100.63,55.15 99.71,54.23 99.71,54.01 v99.66,53.95
  Bottom 1.016: R86.2 R85.1
N$184
  Bottom 0.406: IC8.6 97.04,53.9 98.09,53.9 98.09,51.47 R87.2 97.42,51.47 97.4,45.57 105.35,45.6 105.37,51.47 103.67,51.44 R88.1
N$185
  Bottom 0.406: R87.1 94.53,53.14 95.8,53.14 95.8,56.1 IC8.7 95.77,56.11 91.48,56.11 91.48,64.06 R91.2
N$186  (via drill 0.6 pad 0.81)
  Top 0.813: v104.97,38.82 116.32,38.82 v116.32,38.84
  Bottom 0.406: R90.1 100.88,48.62 R88.2 103.47,48.62 103.47,48.37 | 102.45,48.82 102.35,48.82 102.35,53.62 106.11,53.62 106.11,44 104.92,44 104.92,38.79
  Bottom 0.813: 104.92,38.79 104.97,38.79 v104.97,38.82 | v116.32,38.84 118.46,38.84 T8.E
  Bottom 1.016: T8.E 118.56,38.82 118.56,38.66 | R88.2 100.9,48.75 100.9,48.82 102.45,48.82
N$187
  Bottom 1.016: R89.2 121,34.93 T8.C
N$188
  Bottom 0.406: R92.1 97.04,57.84 IC8.9 97.04,63.96 98.24,63.96 98.24,65.66 C16.2
N$189
  Bottom 0.406: R92.2 93.39,60.69 93.39,60 95.85,60 95.85,61.93 IC8.8 95.75,61.93 C15.2 95.72,65.66 95.72,67.16 100.14,67.16 100.14,70.52 104.64,70.52 R93.2
N$190
  Bottom 1.016: R91.1 93.21,66.91 93.21,68.66 C15.1 C16.1
N$191
  Bottom 0.406: R93.1 101.74,69.02 R94.2 102.12,65.69 IC8.13
N$192
  Bottom 0.406: IC8.14 103.42,61.93 103.42,65.69 R94.1
  Bottom 0.61: 135.22,75.57 110.15,75.57 110.15,68.64 107.23,68.64 107.23,65.56 104.59,65.56 R94.1
  Bottom 0.813: R95.2 135.22,35.51 135.22,75.57
N$193
  Bottom 0.61: 130.44,69.04 130.27,69.04 130.27,72.67
  Bottom 1.016: LED121.A 128.69,50.75 128.69,53.17 130.44,53.17 130.44,69.04 | 130.27,72.67 130.47,72.67 130.47,73.51 113.25,73.51 113.25,54.77 113.35,54.77 113.35,43.13 112.61,43.13 112.61,42.65 112.06,42.65 112.06,30.56 111.44,30.56 LED120.K
N$194
  Bottom 0.61: 131.16,33.43 130.19,33.43 130.19,27.74
  Bottom 1.016: LED121.K 131.16,50.75 131.16,33.43 | 130.19,27.74 131.47,27.74 LED122.A
N$195
  Bottom 1.016: LED122.K 128.9,10.68 128.9,6.51 154.96,6.51 154.96,72.5 148.93,72.5 LED123.A
N$196
  Bottom 1.016: LED123.K 153.46,70.74 153.46,30.66 151.46,30.66 LED124.A
N$197
  Bottom 1.016: LED125.A 148.94,30.72 LED124.K R95.1
N$198
  Bottom 0.61: 151.5,26.67 150.23,26.67 150.23,33.2
  Bottom 1.016: 151.48,50.7 LED126.A 151.45,33.2 150.23,33.2 | LED125.K 151.5,10.75 151.5,26.67
N$199
  Bottom 0.61: 129.96,13.72 130.22,13.72 130.22,7.68 147.44,7.68 147.49,43.26
  Bottom 1.016: LED127.A 128.77,30.69 128.77,25.35 129.96,25.35 129.96,13.72 | 147.49,43.26 148.91,43.34 LED126.K
N$200
  Bottom 1.016: 131.44,70.69 LED128.A 133.14,70.69 133.14,30.84 131.44,30.84 LED127.K
N$201
  Bottom 1.016: LED129.A 108.75,10.75 108.75,8.46 126.69,8.46 126.69,55.61 128.92,55.61 LED128.K
N$202
  Bottom 0.61: 110.4,34.42 110.18,34.42 110.18,27.21
  Bottom 1.016: 111.42,50.7 LED131.A 111.6,50.7 111.6,44.35 110.4,44.35 110.4,34.42 | 110.18,27.21 111.42,27.21 LED129.K
N$203
  Bottom 0.61: 111.32,55.02 110.15,55.02 110.15,48.04
  Bottom 1.016: LED132.K 111.32,70.74 111.32,55.02 | 110.15,48.04 108.9,48.04 LED120.A
N$204
  Bottom 1.016: LED133.A 107.31,30.69 107.31,50.35 108.91,50.35 LED131.K
N$205
  Bottom 1.016: LED134.K 84.9,10.7 84.9,72.9 108.92,72.9 LED132.A
N$206
  Bottom 0.61: 91.38,33.91 90.19,33.91 90.19,26.12
  Bottom 1.016: LED135.K 91.38,50.72 91.38,33.91 | 90.19,26.12 91.47,26.12 LED134.A
N$207
  Bottom 1.016: LED133.K 87.01,30.59 87.01,70.72 LED136.A
N$208
  Bottom 1.016: R96.2 118.48,46.87 LED130.A
N$209  (via drill 0.6 pad 0.81)
  Top 0.406: v179.66,53.95 v173.31,53.95
  Bottom 0.406: 169.73,57.1 169.73,57.26 R97.1 172.73,53.95 v173.31,53.95 | IC9.3 180.83,56.1 180.83,56.16 180.85,56.16 180.85,55.15 180.63,55.15 179.71,54.23 179.71,54.01 v179.66,53.95
  Bottom 1.016: R98.2 R97.1
N$210
  Bottom 0.406: IC9.6 177.04,53.9 178.09,53.9 178.09,51.47 R99.2 177.42,51.47 177.4,45.57 185.35,45.6 185.37,51.47 183.67,51.44 R100.1
N$211
  Bottom 0.406: R99.1 174.53,53.14 175.8,53.14 175.8,56.1 IC9.7 175.77,56.11 171.48,56.11 171.48,64.06 R103.2
N$212  (via drill 0.6 pad 0.81)
  Top 0.813: v184.97,38.82 196.32,38.82 v196.32,38.84
  Bottom 0.406: R102.1 180.88,48.62 R100.2 183.47,48.62 183.47,48.37 | 182.45,48.82 182.35,48.82 182.35,53.62 186.11,53.62 186.11,44 184.92,44 184.92,38.79
  Bottom 0.813: 184.92,38.79 184.97,38.79 v184.97,38.82 | v196.32,38.84 198.46,38.84 T9.E
  Bottom 1.016: T9.E 198.56,38.82 198.56,38.66 | R100.2 180.9,48.75 180.9,48.82 182.45,48.82
N$213
  Bottom 1.016: R101.2 201,34.93 T9.C
N$214
  Bottom 0.406: R104.1 177.04,57.84 IC9.9 177.04,63.96 178.24,63.96 178.24,65.66 C18.2
N$215
  Bottom 0.406: R104.2 173.39,60.69 173.39,60 175.85,60 175.85,61.93 IC9.8 175.75,61.93 C17.2 175.72,65.66 175.72,67.16 180.14,67.16 180.14,70.52 184.64,70.52 R105.2
N$216
  Bottom 1.016: R103.1 173.21,66.91 173.21,68.66 C17.1 C18.1
N$217
  Bottom 0.406: R105.1 181.74,69.02 R106.2 182.12,65.69 IC9.13
N$218
  Bottom 0.406: IC9.14 183.42,61.93 183.42,65.69 R106.1
  Bottom 0.61: 215.22,75.57 190.15,75.57 190.15,68.64 187.23,68.64 187.23,65.56 184.59,65.56 R106.1
  Bottom 0.813: R107.2 215.22,35.51 215.22,75.57
N$219
  Bottom 0.61: 210.44,69.04 210.27,69.04 210.27,72.67
  Bottom 1.016: LED138.A 208.69,50.75 208.69,53.17 210.44,53.17 210.44,69.04 | 210.27,72.67 210.47,72.67 210.47,73.51 193.25,73.51 193.25,54.77 193.35,54.77 193.35,43.13 192.61,43.13 192.61,42.65 192.06,42.65 192.06,30.56 191.44,30.56 LED137.K
N$220
  Bottom 0.61: 211.16,33.43 210.19,33.43 210.19,27.74
  Bottom 1.016: LED138.K 211.16,50.75 211.16,33.43 | 210.19,27.74 211.47,27.74 LED139.A
N$221
  Bottom 1.016: LED139.K 208.9,10.68 208.9,6.51 234.96,6.51 234.96,72.5 228.93,72.5 LED140.A
N$222
  Bottom 1.016: LED140.K 233.46,70.74 233.46,30.66 231.46,30.66 LED141.A
N$223
  Bottom 1.016: LED142.A 228.94,30.72 LED141.K R107.1
N$224
  Bottom 0.61: 231.5,26.67 230.23,26.67 230.23,33.2
  Bottom 1.016: 231.48,50.7 LED143.A 231.45,33.2 230.23,33.2 | LED142.K 231.5,10.75 231.5,26.67
N$225
  Bottom 0.61: 209.96,13.72 210.22,13.72 210.22,7.68 227.44,7.68 227.49,43.26
  Bottom 1.016: LED144.A 208.77,30.69 208.77,25.35 209.96,25.35 209.96,13.72 | 227.49,43.26 228.91,43.34 LED143.K
N$226
  Bottom 1.016: 211.44,70.69 LED145.A 213.14,70.69 213.14,30.84 211.44,30.84 LED144.K
N$227
  Bottom 1.016: LED146.A 188.75,10.75 188.75,8.46 206.69,8.46 206.69,55.61 208.92,55.61 LED145.K
N$228
  Bottom 0.61: 190.4,34.42 190.18,34.42 190.18,27.21
  Bottom 1.016: 191.42,50.7 LED148.A 191.6,50.7 191.6,44.35 190.4,44.35 190.4,34.42 | 190.18,27.21 191.42,27.21 LED146.K
N$229
  Bottom 0.61: 191.32,55.02 190.15,55.02 190.15,48.04
  Bottom 1.016: LED149.K 191.32,70.74 191.32,55.02 | 190.15,48.04 188.9,48.04 LED137.A
N$230
  Bottom 1.016: LED150.A 187.31,30.69 187.31,50.35 188.91,50.35 LED148.K
N$231
  Bottom 1.016: LED151.K 164.9,10.7 164.9,72.9 188.92,72.9 LED149.A
N$232
  Bottom 0.61: 171.38,33.91 170.19,33.91 170.19,26.12
  Bottom 1.016: LED152.K 171.38,50.72 171.38,33.91 | 170.19,26.12 171.47,26.12 LED151.A
N$233
  Bottom 1.016: LED150.K 167.01,30.59 167.01,70.72 LED153.A
N$234
  Bottom 1.016: R108.2 198.48,46.87 LED147.A
S$2  (via drill 0.6)
  Top 0.406: 9.2,207.27 3.35,207.27
  Top 1.016: 169.27,127.16 v162.51,127.16 | 162.46,207.15 169.11,207.15 169.11,207.17 169.14,207.17
  Bottom 1.016: 3.35,207.27 v3.3,207.27 1.88,207.27 1.88,4.02 162.46,4.02 162.46,125.49 | 162.46,127.16 162.46,207.15 | v162.51,127.16 162.46,127.16 | 162.46,127.16 162.46,125.49 | 162.46,125.49 162.48,125.49 162.48,127.11
S$3
  Top 1.016: 169.14,47.23 162.53,47.23 162.53,47.18
  Bottom 1.016: 162.53,47.18 162.41,47.18 162.41,48.68
S$4  (via drill 0.6)
  other vias: 162.51,47.25
S$5  (via drill 0.6)
  Top 1.016: 82.4,206.99 89.08,206.99 89.08,206.97
  Bottom 1.016: 83.16,4.1 82.27,4.1 v82.27,47.2 82.27,73.37 82.32,73.37 82.32,99.07 82.27,99.07 v82.27,127.16 82.27,140.52 82.4,140.52 82.4,206.99 | 89.08,206.97 89,206.97 89,210.68 88.95,210.68 88.95,210.47
S$6  (via drill 0.6)
  other vias: 82.37,207.05
S$7
  Top 1.016: 89.31,127.14 82.32,127.14
  Bottom 1.016: 82.32,127.14 82.25,127.14 82.25,128.08
S$8
  Top 1.016: 89.21,47.23 82.32,47.23 82.32,47.18
  Bottom 1.016: 82.32,47.18 82.3,47.18 82.3,49.11
S$9
  Top 1.016: 9.37,47.18 1.91,47.18 1.91,47.15
  Bottom 1.016: 1.91,47.15 1.91,49.01
S$10  (via drill 0.6)
  other vias: 1.85,47.18
S$11  (via drill 0.6)
  Top 1.016: 8.97,127.11 1.93,127.11 1.93,127.09
  Bottom 1.016: 1.93,127.09 1.91,127.09 v1.91,127.11 1.91,128.43
S$12  (via drill 0.6)
  other vias: 162.51,207.17
S$13  (via drill 0.6)
  Top 1.016: 15.01,230.77 v15.01,237.37 15.01,237.4 | 95.12,71.18 95.17,71.18 v95.17,77.43 95.17,77.45 | 15.24,78.34 14.96,78.34 14.96,70.93
  Bottom 1.016: 11.2,230.69 11.48,230.69 11.48,230.74 15.01,230.74 15.01,230.77 | 15.01,237.4 79.25,237.4 | 79.25,237.4 173.28,237.4 173.28,237.3 159.23,237.3 159.23,159.14 | 159.23,159.14 159.23,159.12 | 159.23,159.12 101.57,159.17 99.62,159.14 159.23,159.14 | 159.23,159.12 159.23,153.73 159.26,153.73 159.26,77.43 v95.17,77.43 95.17,77.45 | 79.25,237.4 79.25,78.32 15.24,78.32 15.24,78.34 | 14.96,70.93 v14.91,70.93 11.48,70.93 11.48,70.24
S$14  (via drill 0.6)
  other vias: 95.15,71.26
S$15  (via drill 0.6)
  other vias: 174.07,71
S$16  (via drill 0.6)
  Top 1.016: 175.39,150.84 175.39,158.51
  Bottom 1.016: 171.12,150.76 v175.39,150.76 175.39,150.84 | 175.39,158.51 237.8,158.51 237.8,158.53
S$17  (via drill 0.6)
  other vias: 175.36,158.56
S$18  (via drill 0.6)
  Top 1.016: 175.23,231.05 175.23,237.32 | 174.07,79.33 v174.12,79.33 174.12,70.98
  Bottom 1.016: 171.42,230.87 171.4,230.87 171.4,231.02 175.23,231.02 175.23,231.05 | 175.23,237.32 176.48,237.32 176.48,237.27 176.53,237.27 176.53,237.35 | 173.38,237.35 176.53,237.35 | 176.53,237.35 237.85,237.35 237.85,79.39 174.07,79.39 174.07,79.33 | 174.12,70.98 171.32,70.98 171.32,70.55 171.42,70.55 171.42,70.8
S$19  (via drill 0.6)
  other vias: 175.18,230.97
S$20  (via drill 0.6)
  other vias: 175.18,237.37
S$21  (via drill 0.6)
  Top 1.016: v95.89,150.86 v95.89,158.79
  Bottom 1.016: 91.57,150.86 v95.89,150.86 | v95.89,158.79 95.86,158.79 95.86,159.17 101.09,159.17 101.09,159.19
S$22
  Bottom 1.016: 91.34,70.95 91.36,70.95 91.36,70.62 91.44,70.62 91.44,71.23 95.17,71.23
S$23
  Top 1.016: 94.84,231.15 94.84,237.3
  Bottom 1.016: 91.29,230.72 91.39,230.72 91.39,231.15 94.84,231.15
S$24  (via drill 0.6)
  other vias: 94.87,231.18
S$25  (via drill 0.6)
  other vias: 94.82,237.37
S$26  (via drill 0.6)
  other vias: 14.99,230.77
S$27  (via drill 0.6)
  other vias: 15.06,78.39
S$28  (via drill 0.6)
  Top 1.016: 14.96,150.76 15.01,150.76 v15.01,150.81 15.01,158.56
  Bottom 1.016: 11.33,150.71 14.96,150.71 14.96,150.76 | 15.01,158.56 79.27,158.56 79.27,158.53 79.1,158.53
S$29  (via drill 0.6)
  other vias: 14.96,158.56
S$30
  Bottom 1.016: 158.75,83.07 153.49,83.07 153.49,78.04 158.42,78.04 158.42,82.1 154.05,82.1 154.05,78.83 158.06,78.83 158.06,78.78 157.68,78.78 157.68,81.47 154.74,81.47 | 154.61,81.47 154.74,81.47 | 154.74,81.47 154.74,79.77 157.51,79.77 157.51,79.64 157.25,79.64 157.25,81.16 155.73,81.16 155.73,80.6 156.39,80.6 156.39,80.3 155.3,80.3 155.3,80.17 157.2,80.17 157.2,80.55
S$31
  Bottom 1.016: 162.74,83.2 168,83.2 168,77.53 163.25,77.53 | 162.76,77.53 163.25,77.53 | 163.25,77.53 163.25,82.36 163.93,82.36 163.93,77.91 164.67,77.91 164.67,82.89 165.48,82.89 165.48,77.91 166.32,77.91 166.32,82.53 167.18,82.53 167.18,77.73 166.95,77.73 166.95,80.12
VCC  (via drill 0.6 pad 0.81)
  Top 0.406: v9.12,207.15 9.17,207.1 v19.2,207.1 36.12,207.1 v36.2,207.17
  Bottom 0.406: 19.63,216.37 19.63,216.1 IC1.4 19.58,215.58 18.67,214.67 18.67,213.19 19.15,212.71 19.15,207.15 v19.2,207.1 | v9.12,207.15 9.12,210.54 LED5.A | v36.2,207.17 35.41,207.17 35.15,207.43
  Bottom 1.016: 8.76,210.96 8.76,210.72 LED5.A 8.93,214.41 R1.2 | R5.1 35.15,194.93 35.15,207.43 35.15,209.71 R13.1 | R13.1
VCC1  (via drill 0.6 pad 0.81)
  Top 0.406: v89.12,207.15 89.17,207.1 v99.2,207.1 116.12,207.1 v116.2,207.17
  Bottom 0.406: 99.63,216.37 99.63,216.1 IC2.4 99.58,215.58 98.67,214.67 98.67,213.19 99.15,212.71 99.15,207.15 v99.2,207.1 | v89.12,207.15 89.12,210.54 LED33.A | v116.2,207.17 115.41,207.17 115.15,207.43
  Bottom 1.016: 88.76,210.96 88.76,210.72 LED33.A 88.93,214.41 R9.2 | R17.1 115.15,194.93 115.15,207.43 115.15,209.71 R24.1 | R24.1
VCC2  (via drill 0.6 pad 0.81)
  Top 0.406: v169.12,207.15 169.17,207.1 v179.2,207.1 196.12,207.1 v196.2,207.17
  Bottom 0.406: 179.63,216.37 179.63,216.1 IC3.4 179.58,215.58 178.67,214.67 178.67,213.19 179.15,212.71 179.15,207.15 v179.2,207.1 | v169.12,207.15 169.12,210.54 LED50.A | v196.2,207.17 195.41,207.17 195.15,207.43
  Bottom 1.016: 168.76,210.96 168.76,210.72 LED50.A 168.93,214.41 R25.2 | R29.1 195.15,194.93 195.15,207.43 195.15,209.71 R36.1 | R36.1
VCC3  (via drill 0.6 pad 0.81)
  Top 0.406: v9.12,127.15 9.17,127.1 v19.2,127.1 36.12,127.1 v36.2,127.17
  Bottom 0.406: 19.63,136.37 19.63,136.1 IC4.4 19.58,135.58 18.67,134.67 18.67,133.19 19.15,132.71 19.15,127.15 v19.2,127.1 | v9.12,127.15 9.12,130.54 LED67.A | v36.2,127.17 35.41,127.17 35.15,127.43
  Bottom 1.016: 8.76,130.96 8.76,130.72 LED67.A 8.93,134.41 R37.2 | R41.1 35.15,114.93 35.15,127.43 35.15,129.71 R48.1 | R48.1
VCC4  (via drill 0.6 pad 0.81)
  Top 0.406: v89.12,127.15 89.17,127.1 v99.2,127.1 116.12,127.1 v116.2,127.17
  Bottom 0.406: 99.63,136.37 99.63,136.1 IC5.4 99.58,135.58 98.67,134.67 98.67,133.19 99.15,132.71 99.15,127.15 v99.2,127.1 | v89.12,127.15 89.12,130.54 LED84.A | v116.2,127.17 115.41,127.17 115.15,127.43
  Bottom 1.016: 88.76,130.96 88.76,130.72 LED84.A 88.93,134.41 R49.2 | R53.1 115.15,114.93 115.15,127.43 115.15,129.71 R60.1 | R60.1
VCC5  (via drill 0.6 pad 0.81)
  Top 0.406: v169.12,127.15 169.17,127.1 v179.2,127.1 196.12,127.1 v196.2,127.17
  Bottom 0.406: 179.63,136.37 179.63,136.1 IC6.4 179.58,135.58 178.67,134.67 178.67,133.19 179.15,132.71 179.15,127.15 v179.2,127.1 | v169.12,127.15 169.12,130.54 LED101.A | v196.2,127.17 195.41,127.17 195.15,127.43
  Bottom 1.016: 168.76,130.96 168.76,130.72 LED101.A 168.93,134.41 R61.2 | R65.1 195.15,114.93 195.15,127.43 195.15,129.71 R72.1 | R72.1
VCC6  (via drill 0.6 pad 0.81)
  Top 0.406: v9.12,47.15 9.17,47.1 v19.2,47.1 36.12,47.1 v36.2,47.17
  Bottom 0.406: 19.63,56.37 19.63,56.1 IC7.4 19.58,55.58 18.67,54.67 18.67,53.19 19.15,52.71 19.15,47.15 v19.2,47.1 | v9.12,47.15 9.12,50.54 LED118.A | v36.2,47.17 35.41,47.17 35.15,47.43
  Bottom 1.016: 8.76,50.96 8.76,50.72 LED118.A 8.93,54.41 R73.2 | R77.1 35.15,34.93 35.15,47.43 35.15,49.71 R84.1 | R84.1
VCC7  (via drill 0.6 pad 0.81)
  Top 0.406: v89.12,47.15 89.17,47.1 v99.2,47.1 116.12,47.1 v116.2,47.17
  Bottom 0.406: 99.63,56.37 99.63,56.1 IC8.4 99.58,55.58 98.67,54.67 98.67,53.19 99.15,52.71 99.15,47.15 v99.2,47.1 | v89.12,47.15 89.12,50.54 LED135.A | v116.2,47.17 115.41,47.17 115.15,47.43
  Bottom 1.016: 88.76,50.96 88.76,50.72 LED135.A 88.93,54.41 R85.2 | R89.1 115.15,34.93 115.15,47.43 115.15,49.71 R96.1 | R96.1
VCC8  (via drill 0.6 pad 0.81)
  Top 0.406: v169.12,47.15 169.17,47.1 v179.2,47.1 196.12,47.1 v196.2,47.17
  Bottom 0.406: 179.63,56.37 179.63,56.1 IC9.4 179.58,55.58 178.67,54.67 178.67,53.19 179.15,52.71 179.15,47.15 v179.2,47.1 | v169.12,47.15 169.12,50.54 LED152.A | v196.2,47.17 195.41,47.17 195.15,47.43
  Bottom 1.016: 168.76,50.96 168.76,50.72 LED152.A 168.93,54.41 R97.2 | R101.1 195.15,34.93 195.15,47.43 195.15,49.71 R108.1 | R108.1

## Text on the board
Top: gnd | gnd | VCC | VCC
